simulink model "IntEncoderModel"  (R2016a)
settings: Solver=VariableStepAuto  StartTime=0.0  StopTime=10.0  RelTol=1e-3
undefined symbols (not defined in the file): High, torque, VEX
libraries: vexarmcortexlib x3

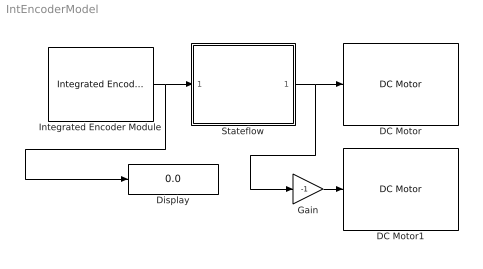
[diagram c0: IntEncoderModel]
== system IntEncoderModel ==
  DC Motor : vexarmcortexlib/DC Motor  motor=3  scaleFactor=1/13.5  SimulationOut=off
  DC Motor1 : vexarmcortexlib/DC Motor  motor=7  scaleFactor=1/13.5  SimulationOut=off
  Display : Display
  Gain : Gain  Gain=-1
  Integrated Encoder Module : vexarmcortexlib/Integrated Encoder Module  motorType=VEX 393 (High torque)  seqNumI2C=0  resetOption=No reset  rotVelocity=off  inputPortSim=off  SampleTime=0.2
  Stateflow : Stateflow chart  TreatAsAtomicUnit=on
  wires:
  Integrated Encoder Module/1 -> Display/1, Stateflow/1(inshaft)
  Stateflow/1(speed) -> Gain/1, DC Motor/1
  Gain/1 -> DC Motor1/1

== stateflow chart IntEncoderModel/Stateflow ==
  state Drive_Forward
    during:
    speed =-30;
  state Stop
    during:
    speed =0;
  (default) -> Drive_Forward : {speed = 0;}
  Drive_Forward -> Stop : [inshaft > 1800]
  data: inshaft input; speed output
